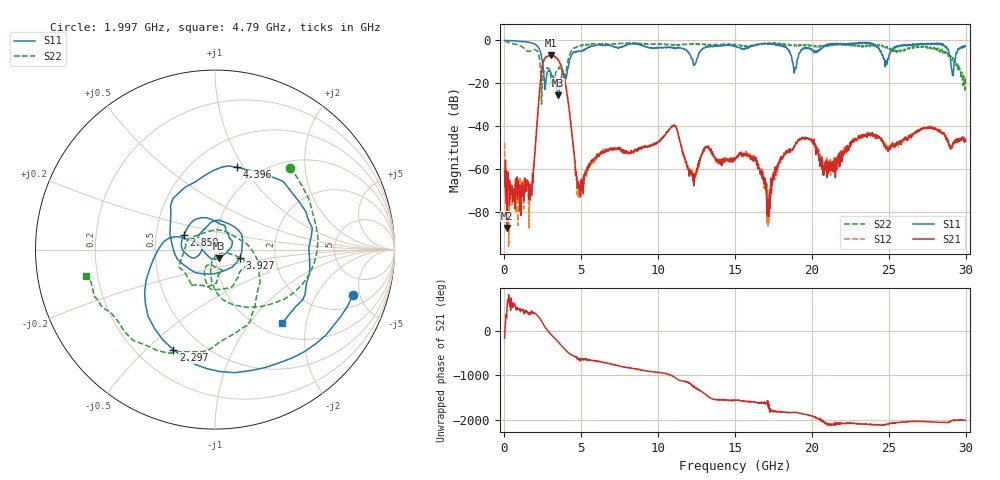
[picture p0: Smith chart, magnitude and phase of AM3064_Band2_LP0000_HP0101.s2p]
# Hz S DB R 50.0
!freq dBS11 angS11 dBS21 angS21 dBS12 angS12 dBS22 angS22
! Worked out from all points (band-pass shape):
!   1600 points, 10 MHz to 29.98 GHz, reference 50 ohm
!   highest |S21| = -6.99 dB at 3.046 GHz (marker M1); lowest = -87.3 dB at 159.9 MHz (marker M2)
!   |S21| within 3 dB of the highest: 2.533 GHz to 3.556 GHz (1.023 GHz wide, 33.6 % of centre)
!   lowest |S11| = -25.6 dB at 3.478 GHz (marker M3), VSWR 1.11, Z = 51.8 - j5.06 ohm
!   |S11| at or under -10 dB: 2.463 GHz to 4.207 GHz (1.744 GHz wide, 52.3 % of centre); 18.73 GHz to 19.02 GHz (290.2 MHz wide, 1.54 % of centre); 29.02 GHz to 29.25 GHz (227.8 MHz wide, 0.782 % of centre)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
!   |S22| runs from -29.7 to -0.2 dB; largest |S21 - S12| = 0.017
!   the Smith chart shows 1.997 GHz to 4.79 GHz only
!   S11 on the Smith chart (normalised r, x): 1.997 GHz: 2.90, -4.29; 2.297 GHz: 0.35, -0.61; 2.859 GHz: 0.70, +0.12; 3.927 GHz: 1.32, -0.12; 4.396 GHz: 0.79, +0.93; 4.79 GHz: 1.23, -1.47
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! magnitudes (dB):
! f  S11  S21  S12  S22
! 10 MHz  0.0  -61.0  -47.7  -0.2
! 159.9 MHz  -0.1  -87.3  -65.2  -0.7
! 1.659 GHz  -1.0  -74.1  -70.3  -5.0
! 1.997 GHz  -1.8  -50.3  -50.7  -4.2
! 2.297 GHz  -4.4  -22.5  -22.5  -9.8
! 2.859 GHz  -14.4  -7.2  -7.2  -13.0
! 3.046 GHz  -15.6  -7.0  -7.0  -18.7
! 3.478 GHz  -25.6  -8.9  -9.0  -13.5
! 3.927 GHz  -16.7  -18.6  -18.5  -18.9
! 4.396 GHz  -6.5  -43.8  -43.7  -4.6
! 4.79 GHz  -5.1  -65.9  -68.3  -2.7
! 5.015 GHz  -5.0  -68.1  -64.5  -2.5
! 10 GHz  -3.4  -47.2  -47.3  -1.7
! 11.09 GHz  -3.9  -39.8  -39.7  -1.9
! 12.31 GHz  -11.7  -62.4  -65.8  -1.6
! 15 GHz  -2.6  -55.5  -55.4  -1.9
! 17.2 GHz  -1.6  -82.2  -71.4  -1.7
! 18.19 GHz  -2.4  -53.5  -52.2  -1.8
! 19.99 GHz  -4.2  -46.8  -46.8  -2.2
! 20.89 GHz  -2.1  -59.5  -61.0  -2.9
! 25 GHz  -8.2  -50.2  -48.8  -3.1
! 29.98 GHz  -2.5  -47.0  -46.4  -17.3
